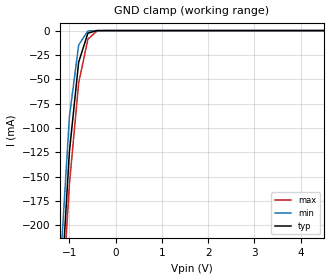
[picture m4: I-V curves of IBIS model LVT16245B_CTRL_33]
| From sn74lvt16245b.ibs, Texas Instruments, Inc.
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|  Model LVT16245B Input CTRL_33
[Model]   LVT16245B_CTRL_33
Model_type  Input
Polarity   Inverting
Vinl = 0.8V
Vinh = 2.0V
| variable   typ   min   max
C_comp   4p   NA   NA
[Temperature Range]   40   -25   100
| Ambient Temperature   25   -40   85
[Voltage range]   3.3   3.0   3.6
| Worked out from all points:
|   GND clamp passes 1 mA (typ) near -0.48 V on its own axis
[GND Clamp]
|   Voltage   V(typ)   V(min)   V(max)
-5V       -4.237A    -4.661A    -3.845A
-1.2V     -285.1mA   -245.1mA   -312mA
-1V       -124.4mA   -88.53mA   -157.9mA
-800mV    -32.48mA   -14.85mA   -53.9mA
-600mV    -2.6mA     -353.7uA   -8.777mA
-400mV    -8.779uA   -387.8nA   -243.3uA
5V        493.8pA    2.701uA    646.3pA
